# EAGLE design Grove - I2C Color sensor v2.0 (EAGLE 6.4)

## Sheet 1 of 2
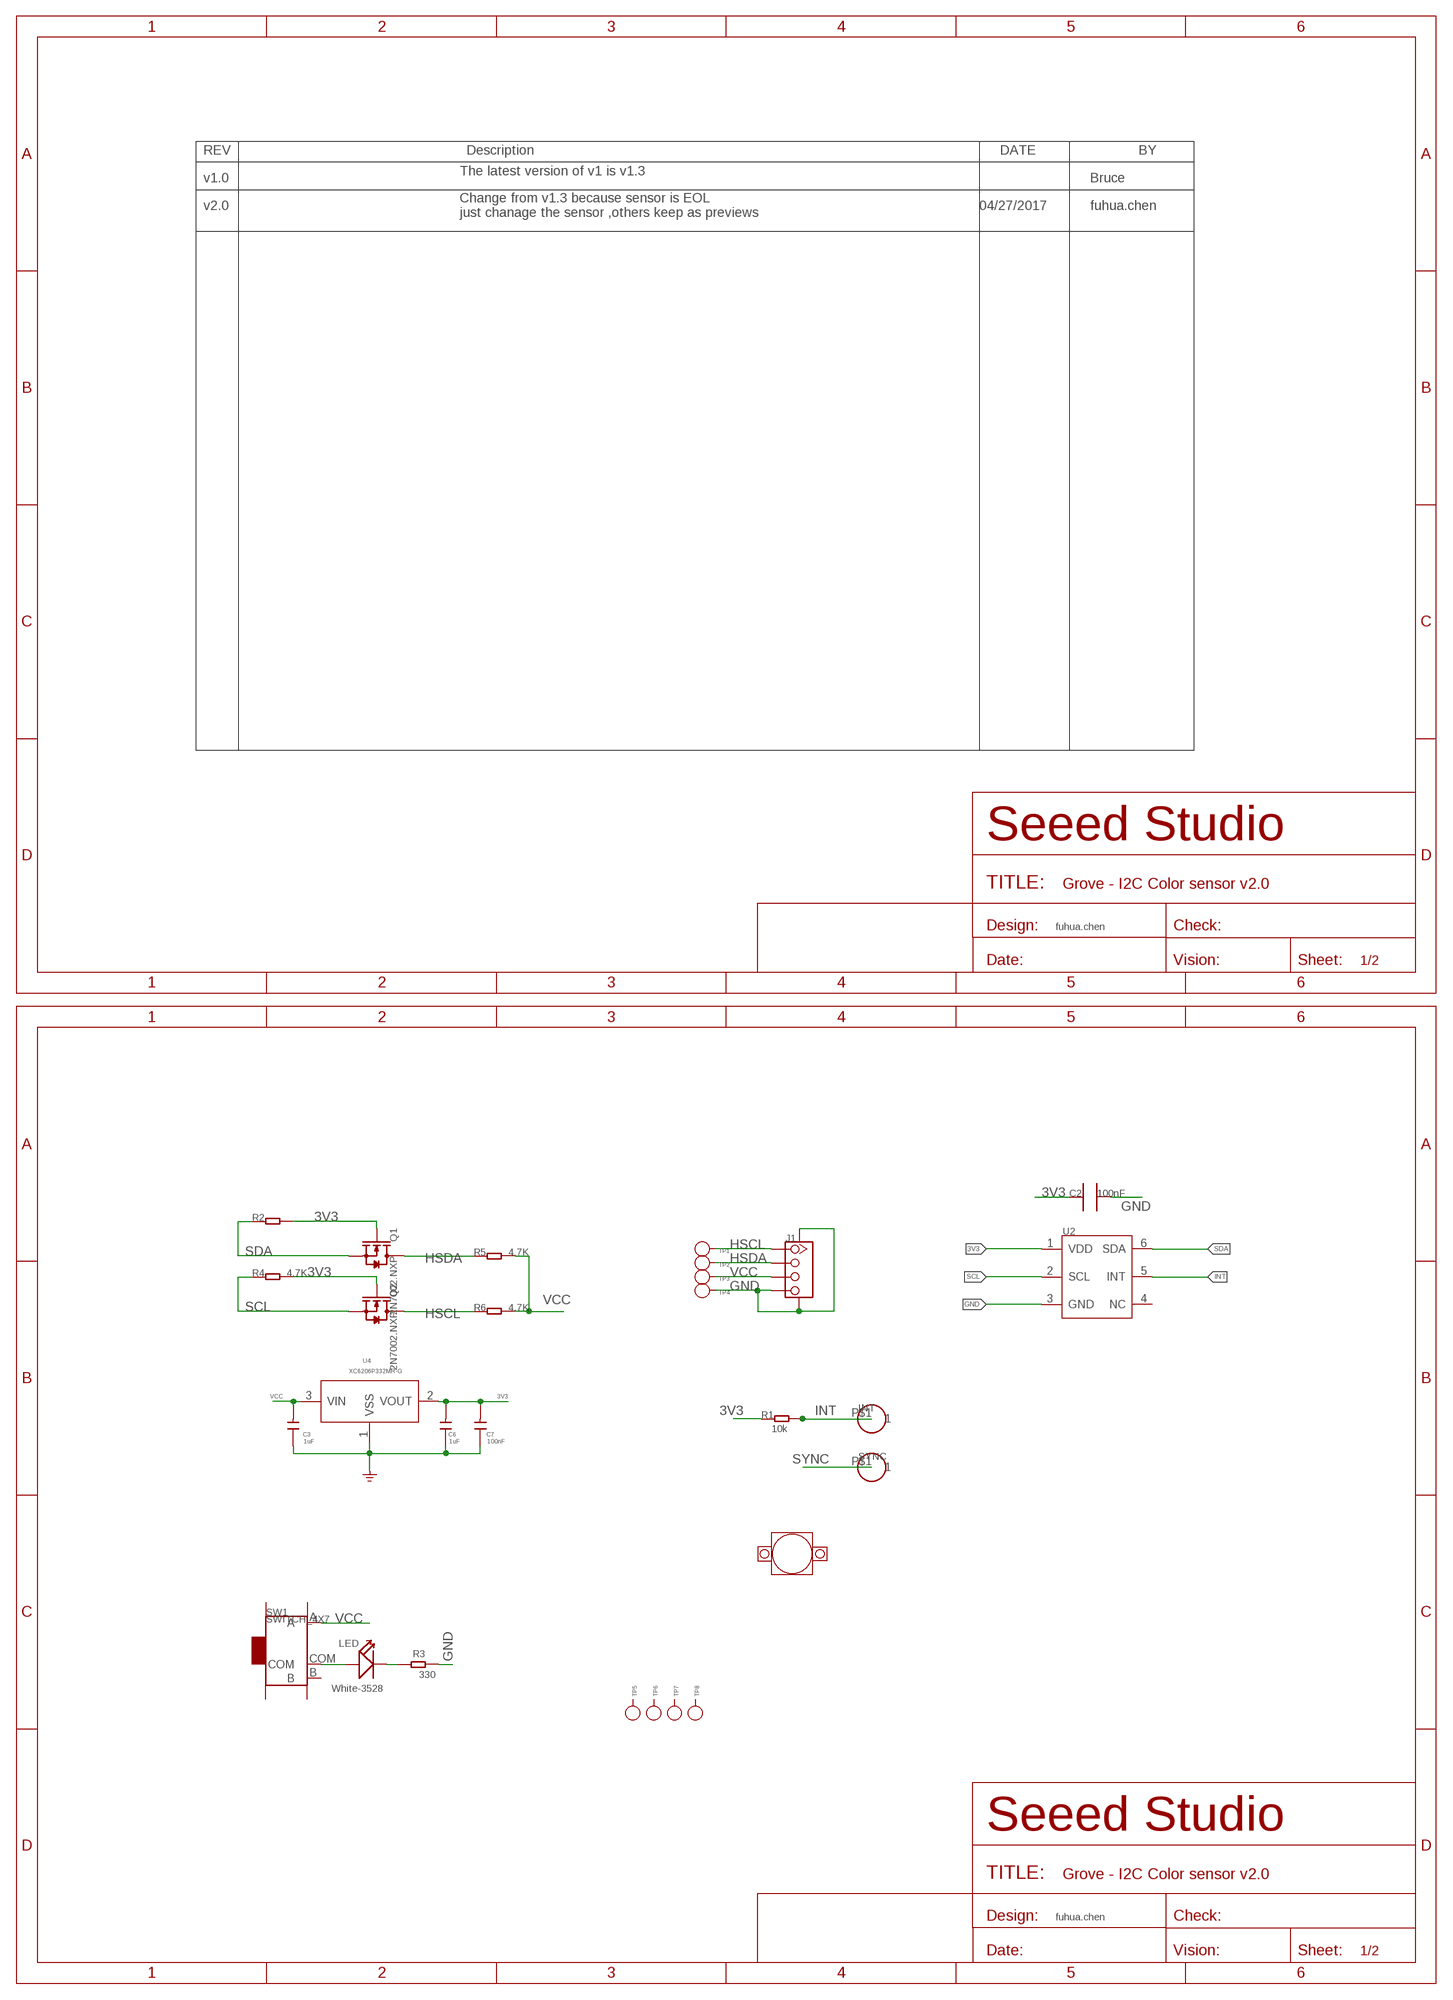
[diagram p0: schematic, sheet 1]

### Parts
C2  100nF  C0603_S  [0603_S]
C3  1uF  C-0603  [C0603]
C6  1uF  C-0603  [C0603]
C7  100nF  C-0603  [C0603]
INT  CK_1X132  [CK_1X1]
J1  TWIG-4P-2.0-SMD-FEMALE-REINFORCE'DD'  [4P-SMD-2.0]
LED  White-3528  007-LED1.6*2.7  [LED1210]
Q1  2N7002.NXP  MOSFET-N'SOT23'  [SOT23]
Q2  2N7002.NXP  MOSFET-N'SOT23'  [SOT23]
R1  10k  R-0603  [R0603]
R2  R-0603  [R0603]
R3  330  R-0603  [R0603]
R4  4.7K  R-0603  [R0603]
R5  4.7K  R-0603  [R0603]
R6  4.7K  R-0603  [R0603]
SW1  SWITCH_4X7  [4*8_SW]
SYNC  CK_1X132  [CK_1X1]
TP1  PAD-TEST-POINT'4545'  [TP_4545]
TP2  PAD-TEST-POINT'4545'  [TP_4545]
TP3  PAD-TEST-POINT'4545'  [TP_4545]
TP4  PAD-TEST-POINT'4545'  [TP_4545]
TP5  PAD-TEST-POINT'4545'  [TP_4545]
TP6  PAD-TEST-POINT'4545'  [TP_4545]
TP7  PAD-TEST-POINT'4545'  [TP_4545]
TP8  PAD-TEST-POINT'4545'  [TP_4545]
U2  SENSOR-TCS34725FN  [DFN6-0.65-2.4X2X0.65MM]
U3  LENS_HOOD  [LENS_HOOD]
U4  XC6206P332MR-G  XC6206MR  [SOT23]

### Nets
3V3: C2.1 C6.2 C7.2 Q1.1(G) Q2.1(G) R1.1 R2.2 R4.2 U2.1(VDD) U4.2(VOUT)
GND: C2.2 C3.1 C6.1 C7.1 J1.4 J1.SS1 J1.SS2 R3.1 TP4.T U2.3(GND) U4.1(VSS)
HSCL: J1.1 Q2.3(D) R6.1 TP1.T
HSDA: J1.2 Q1.3(D) R5.1 TP2.T
INT: INT.P$1 R1.2 U2.5(INT)
N$2: LED.1(+) SW1.COM
N$5: LED.2(-) R3.2
SCL: Q2.2(S) R4.1 U2.2(SCL)
SDA: Q1.2(S) R2.1 U2.6(SDA)
SYNC: SYNC.P$1
VCC: C3.2 J1.3 R5.2 R6.2 SW1.A TP3.T U4.3(VIN)
Unconnected: SW1.B SW1.SS1 SW1.SS2 SW1.SS3 SW1.SS4 TP5.T TP6.T TP7.T TP8.T U2.4(NC)

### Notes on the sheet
- The latest version of v1 is v1.3
- v1.0 | Bruce
- v2.0 | 04/27/2017 | fuhua.chen
- Change from v1.3 because sensor is EOL
  just chanage the sensor ,others keep as previews
- fuhua.chen
- fuhua.chen

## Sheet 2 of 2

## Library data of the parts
C2 = CPT_SMD:C0603
C3 C6 C7 = Discrete:C*: Ceramic Capacitors
INT SYNC = CONNECTER1:CK_1X1
J1 = Connector:TWIG-4P-2.0-SMD-FEMALE-REINFORCE
LED = Discrete:007-LED*
Q1 Q2 = Discrete:MOSFET-N: IRLL014: http://www.vishay.com/docs/91319/sihll014.pdf
R1-R6 = Discrete:R*
SW1 = CPT_SMD:SWITCH
TP1-TP8 = Discrete:PAD-TEST-POINT; PARTNO: DNP
U2 = Discrete-new:SENSOR-TCS34725FN: 314990022
U3 = machine:LENS_HOOD
U4 = IC:XC6206: LOW ESR Cap.Compatible Positive Voltage Regulators

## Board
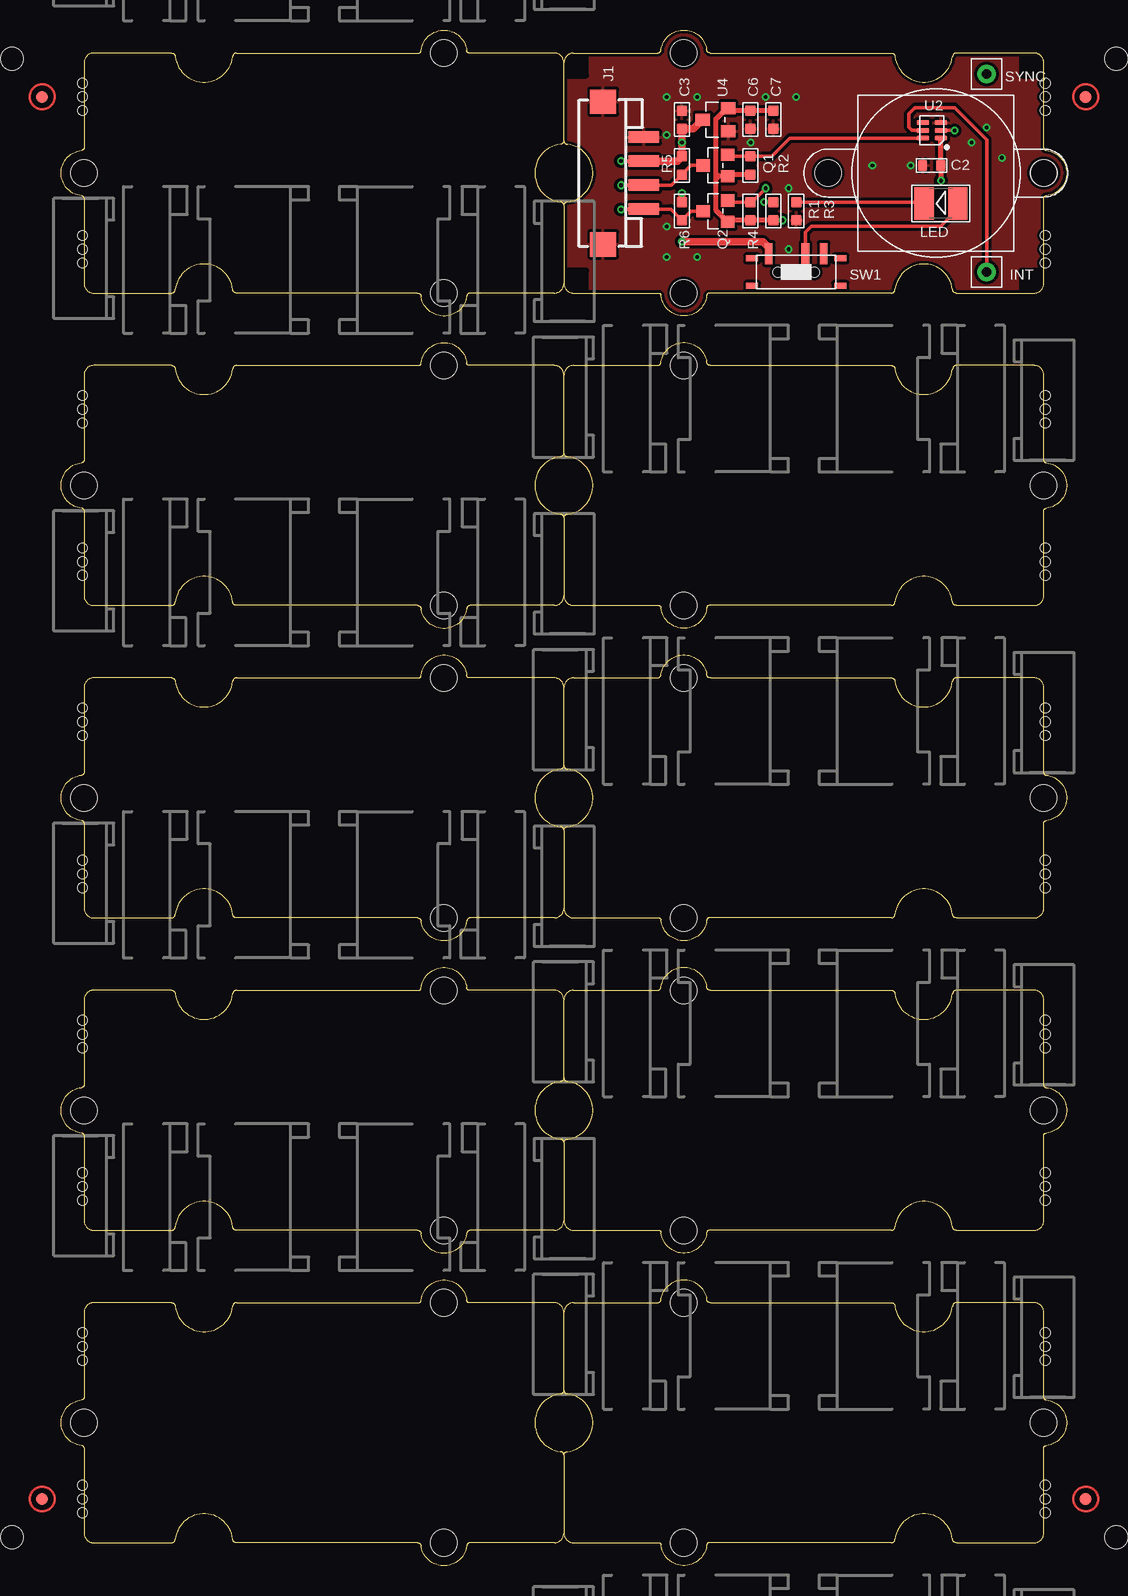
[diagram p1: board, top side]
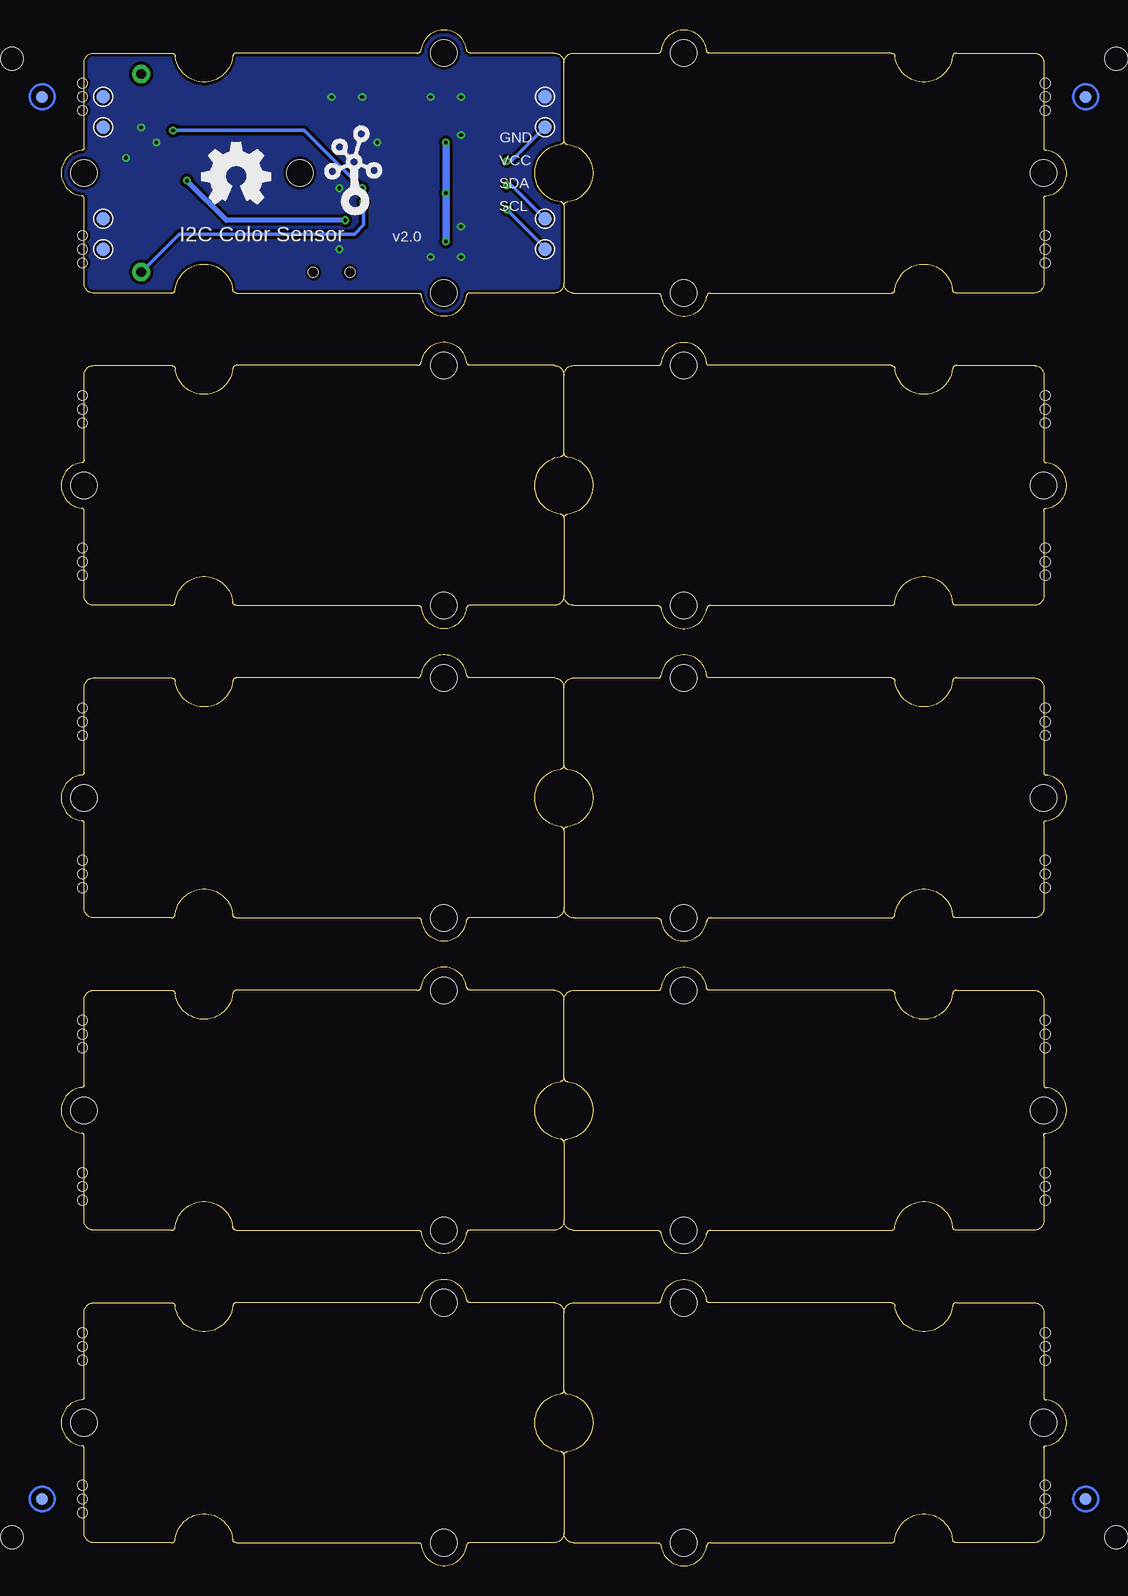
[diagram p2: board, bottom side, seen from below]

Size 83.82 x 127.98 mm. Coordinates in mm from the lower left corner, seen from the top.
Copper layers (1*16): Top 0.035mm / dielectric 1.5mm / Bottom 0.035mm
Design rules "SeeedStudio_2layer_DRU_no_angle_20140221 *": minimum track width 6mil, minimum drill 12mil, track to track 6mil, track to pad 6mil, pad to pad 6mil, via to via 6mil, smd to smd 0mil, copper to edge 10mil, drill to drill 10mil, minimum pad ring 10mil, minimum via ring 6mil, stop-mask expansion 2mil, vias tented up to drill 100mil, thermal gap 10mil
Holes 0.8 mm at 82.04,4.43 82.04,6.71 82.04,5.57 82.04,17.13 82.04,19.41 82.04,18.27 82.04,30.46 82.04,32.75 82.04,31.61 82.04,43.16 82.04,45.45 82.04,44.31 82.04,56.5 82.04,58.78 82.04,57.64 82.04,69.2 82.04,71.48 82.04,70.34 82.04,82.53 82.04,84.82 82.04,83.68 82.04,95.23 82.04,97.52 82.04,96.38 82.04,108.57 82.04,110.85 82.04,109.71 82.04,121.27 82.04,123.55 82.04,122.41 1.78,6.71 1.78,4.43 1.78,5.57 1.78,19.41 1.78,17.13 1.78,18.27 1.78,32.75 1.78,30.46 1.78,31.61 1.78,45.45 1.78,43.16 1.78,44.31 1.78,58.78 1.78,56.5 1.78,57.64 1.78,71.48 1.78,69.2 1.78,70.34 1.78,84.82 1.78,82.53 1.78,83.68 1.78,97.52 1.78,95.23 1.78,96.38 1.78,110.85 1.78,108.57 1.78,109.71 1.78,123.55 1.78,121.27 1.78,122.41
Holes 1.91 mm at 87.95,125.59 -4.13,125.59 -4.13,2.4 87.95,2.4

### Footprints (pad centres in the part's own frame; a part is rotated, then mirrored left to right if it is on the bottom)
0603_S = smd 0.762 x 0.889: 1 -0.762,0; 2 0.762,0
C0603 = smd 0.889 x 0.889: 1 -0.762,0; 2 0.762,0
CK_1X1 = drill 0.813 pad 1.524: P$1 0,0
4P-SMD-2.0 = smd 0.965 x 2.54: 1 -3,0; 2 -1,0; 3 1,0; 4 3,0 | smd 2.032 x 2.184: SS1 -5.946,3.4; SS2 5.946,3.4
LED1210 = smd 1.6 x 2.7: 1 -1.4,0; 2 1.4,0
ROUND-MARK-1.0 = smd 1.016 x 1.016: P$1 0,0
SOT23 = smd 1.016 x 1.143: 1 -0.889,-1.016; 2 0.889,-1.016; 3 0,1.016
R0603 = smd 0.889 x 0.889: 1 -0.762,0; 2 0.762,0
4*8_SW = smd 1.778 x 0.635: A 1.524,2.286; B 1.524,-2.286; COM 1.524,-0.762 | smd 0.508 x 1.016: SS1 -1.143,-3.683; SS2 1.143,-3.683; SS3 1.143,3.683; SS4 -1.143,3.683 | hole 0.813: 0,-1.524; 0,1.524
TP_4545 = smd 1.143 x 1.143: T 0,0
GROVE-TEST-PLATFORM = hole 2.2: -10,-10; -10,10; 20,0
DFN6-0.65-2.4X2X0.65MM = smd 1 x 0.4: 1 -0.75,0.65; 2 -0.75,0; 3 -0.75,-0.65; 4 0.75,-0.65; 5 0.75,0; 6 0.75,0.65
LENS_HOOD = hole 2.2: 9,0; -9,0
SOT23' = smd 1.016 x 1.2: 1 -0.95,-1.06; 2 0.95,-1.06; 3 0,1.06

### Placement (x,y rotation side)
C2  72.58,116.7 180 top
C3  51.75,120.51 270 top
C6  57.47,120.51 90 top
C7  59.37,120.51 90 top
INT  77.15,107.81 270 top
J1  48.58,116.06 90 top
LED  73.34,113.52 180 top
P1  [ROUND-MARK-1.0]  85.41,122.41 180 top
P2  [ROUND-MARK-1.0]  -1.59,122.41 180 top
P3  [ROUND-MARK-1.0]  85.41,5.57 180 top
P4  [ROUND-MARK-1.0]  -1.59,5.57 180 top
P5  [ROUND-MARK-1.0]  85.41,122.41 180 bottom
P6  [ROUND-MARK-1.0]  -1.59,122.41 180 bottom
P7  [ROUND-MARK-1.0]  -1.59,5.57 180 bottom
P8  [ROUND-MARK-1.0]  85.41,5.57 180 bottom
Q1  54.55,116.7 90 top
Q2  54.55,112.89 90 top
R1  59.37,112.89 90 top
R2  57.47,116.7 270 top
R3  61.28,112.89 90 top
R4  57.47,112.89 270 top
R5  51.75,116.7 90 top
R6  51.75,112.89 90 top
SW1  61.28,107.81 90 top
SYNC  77.15,124.32 270 top
TP1  43.5,109.71 180 bottom
TP2  43.5,112.25 180 bottom
TP3  43.5,119.87 180 bottom
TP4  43.5,122.41 180 bottom
TP5  80.33,112.25 180 bottom
TP6  80.33,119.87 180 bottom
TP7  80.33,122.41 180 bottom
TP8  80.33,109.71 180 bottom
U1  [GROVE-TEST-PLATFORM]  21.91,90.03 180 top
U2  72.58,119.62 180 top
U3  72.92,116.06 180 top
U4  XC6206P332MR-G  [SOT23']  54.55,120.51 90 top
U5  [GROVE-TEST-PLATFORM]  61.91,90.03 0 top
U6  [GROVE-TEST-PLATFORM]  21.91,63.99 180 top
U7  [GROVE-TEST-PLATFORM]  61.91,63.99 0 top
U8  [GROVE-TEST-PLATFORM]  21.91,37.96 180 top
U9  [GROVE-TEST-PLATFORM]  61.91,37.96 0 top
U10  [GROVE-TEST-PLATFORM]  61.91,11.92 0 top
U11  [GROVE-TEST-PLATFORM]  21.91,11.92 180 top
U12  [GROVE-TEST-PLATFORM]  21.91,116.06 180 top
U13  [GROVE-TEST-PLATFORM]  61.91,116.06 0 top
U$1  [TWIGLOGO]  59.37,113.52 0 bottom
U$2  [GROVE-TEST-PLATFORM]  61.91,116.06 0 top
U$3  [OSHW_FILLX200_NOTEXT]  72.07,113.52 0 bottom

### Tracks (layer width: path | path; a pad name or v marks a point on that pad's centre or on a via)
3V3  (via drill 0.3 pad 0.64)
  Top 0.406: C7.2 C6.2 | C6.2 55.8,121.27 U4.2 | R2.2 55.69,115.93 Q1.1 54.8,115.81 | C6.2 55.31,121.27 54.55,120.51 54.55,116.06 | 54.55,116.06 54.55,115.81 | 54.55,115.81 54.55,115.55 | 54.55,115.55 54.55,113.01 Q2.1 55.69,112.12 R4.2 R1.1 v60.14,112.12 | 54.8,115.81 54.55,115.81 | 54.8,115.81 54.55,116.06 | 54.8,115.81 54.55,115.55 | v73.34,115.43 C2.1 73.34,118.96 U2.1
  Bottom 0.406: v60.14,112.12 70.04,112.12 v73.34,115.43
GND  (via drill 0.3 pad 0.64)
  other vias: 57.47,118.6 53.02,122.41 60.64,109.71 50.48,122.41 50.48,119.24 50.48,111.62 58.74,122.41 60.64,114.79 61.28,122.41 53.02,109.08 50.48,109.08 75.88,118.6 77.15,119.87 78.42,117.33 70.8,116.7 67.63,116.7
  pour Bottom (isolate 0.254): 41.59,128.76 84.77,128.76 84.77,103.36 41.59,103.36
  pour Top (isolate 0.254): 41.59,128.76 84.77,128.76 84.77,103.36 41.59,103.36
HSCL  (via drill 0.3 pad 0.64)
  Top 0.305: v46.67,113.01 46.72,113.06 J1.1 50.82,113.06 R6.1 52.52,112.89 Q2.3
  Bottom 0.305: v46.67,113.01 46.29,112.63 46.17,112.51 43.5,109.84 TP1.T
HSDA  (via drill 0.3 pad 0.64)
  Top 0.305: v46.67,115.05 46.69,115.06 J1.2 50.88,115.06 51.63,115.81 R5.1 52.52,116.7 Q1.3
  Bottom 0.305: v46.67,115.05 46.29,115.05 TP2.T
INT  (via drill 0.3 pad 0.64)
  Top 0.305: R1.2 v58.61,113.65 | INT.P$1 77.15,118.86 74.49,121.52 71.18,121.52 70.68,121.01 70.68,119.87 70.93,119.62 U2.5
  Bottom 0.305: v58.61,113.65 58.61,111.74 59.37,110.98 73.98,110.98 INT.P$1
N$2
  Top 0.305: LED.1 74.74,113.02 73.34,111.62 62.55,111.62 62.04,111.11 SW1.COM
N$5
  Top 0.305: R3.2 71.82,113.65 LED.2
SCL  (via drill 0.3 pad 0.64)
  Top 0.305: Q2.2 55.69,113.65 R4.1 57.6,113.65 v58.74,114.79 | U2.2 v74.49,119.62
  Bottom 0.305: v58.74,114.79 63.12,119.17 63.18,119.24 63.56,119.62 v74.49,119.62
SDA
  Top 0.305: Q1.2 55.69,117.46 R2.1 59.25,117.46 60.39,118.6 60.52,118.73 60.76,118.97 U2.6
VCC  (via drill 0.3 pad 0.64)
  Top 0.305: J1.3 46.69,117.06 v46.67,117.08
  Top 0.61: J1.3 51.36,117.06 R5.2 v51.75,118.6 C3.2 | 51.75,119.87 C3.2 | C3.2 52.73,119.74 U4.3 | R6.2 v51.75,114.41 | v51.75,110.35 58.48,110.35 58.99,109.84 SW1.A
  Bottom 0.305: v46.67,117.08 46.29,117.08 TP3.T
  Bottom 0.61: v51.75,118.6 51.75,115.05 v51.75,114.41 v51.75,110.35

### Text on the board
bPlace: GND | VCC | SDA | SCL | v2.0 | I2C Color Sensor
